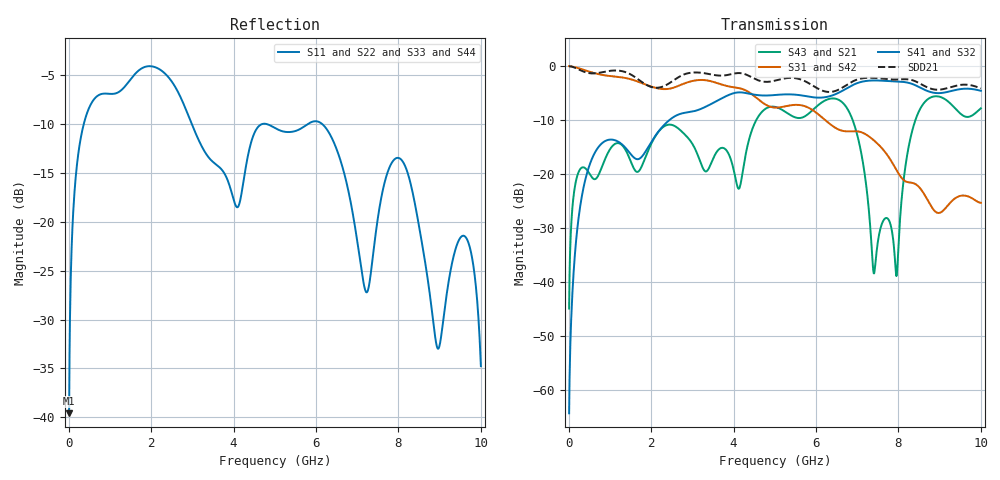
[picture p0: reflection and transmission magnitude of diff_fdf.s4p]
# HZ S RI R 50
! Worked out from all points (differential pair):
!   1000 points, 10 MHz to 10 GHz, reference 50 ohm
!   strongest paths, dB at 10 MHz, 2.51 GHz, 5.01 GHz, 7.51 GHz, 10 GHz:
!     S41: -64.4, -9.6, -5.4, -2.7, -4.6
!     S32: -64.4, -9.6, -5.4, -2.7, -4.6
!     S31: 0.0, -4.1, -7.7, -14.5, -25.3
!     S42: 0.0, -4.1, -7.7, -14.5, -25.3
!     S43: -44.9, -10.9, -7.6, -32.1, -7.8
!     S21: -44.9, -10.9, -7.6, -32.1, -7.8
!   taken as a pair (ports 1,2 in; 3,4 out), SDD21 dB: 0.0, -2.8, -2.7, -2.2, -4.2
!   lowest |S11| = -39.6 dB at 10 MHz (marker M1), VSWR 1.02, Z = 49.9 - j1.05 ohm
!   |S11| at or under -10 dB: 2.984 GHz to 4.713 GHz (1.729 GHz wide, 44.9 % of centre); 4.779 GHz to 5.807 GHz (1.028 GHz wide, 19.4 % of centre); 6.145 GHz to end of sweep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
1e7  -0.000638 -0.0105  0.000355 0.00565  0.9982 -0.0423  9.46e-05 -0.000597
     0.000355 0.00565  -0.000638 -0.0105  9.46e-05 -0.000597  0.9982 -0.0423
     0.9982 -0.0423  9.46e-05 -0.000597  -0.000638 -0.0105  0.000355 0.00565
     9.46e-05 -0.000597  0.9982 -0.0423  0.000355 0.00565  -0.000638 -0.0105
8.4e8  0.1036 0.4391  0.1207 0.0352  -0.8111 0.1555  0.0712 0.184
       0.1207 0.0352  0.1036 0.4391  0.0712 0.184  -0.8111 0.1555
       -0.8111 0.1555  0.0712 0.184  0.1036 0.4391  0.1207 0.0352
       0.0712 0.184  -0.8111 0.1555  0.1207 0.0352  0.1036 0.4391
1.58e9  0.0226 -0.5593  -0.0871 -0.0716  0.7383 0.0631  -0.041 -0.1363
        -0.0871 -0.0716  0.0226 -0.5593  -0.041 -0.1363  0.7383 0.0631
        0.7383 0.0631  -0.041 -0.1363  0.0226 -0.5593  -0.0871 -0.0716
        -0.041 -0.1363  0.7383 0.0631  -0.0871 -0.0716  0.0226 -0.5593
2.47e9  -0.0181 0.5306  0.2865 0.0093  -0.6203 -0.0131  0.00072 0.3223
        0.2865 0.0093  -0.0181 0.5306  0.00072 0.3223  -0.6203 -0.0131
        -0.6203 -0.0131  0.00072 0.3223  -0.0181 0.5306  0.2865 0.0093
        0.00072 0.3223  -0.6203 -0.0131  0.2865 0.0093  -0.0181 0.5306
7.29e9  0.0343 -0.0332  -0.0406 -0.0131  -0.2222 -0.00121  0.039 0.7326
        -0.0406 -0.0131  0.0343 -0.0332  0.039 0.7326  -0.2222 -0.00121
        -0.2222 -0.00121  0.039 0.7326  0.0343 -0.0332  -0.0406 -0.0131
        0.039 0.7326  -0.2222 -0.00121  -0.0406 -0.0131  0.0343 -0.0332
7.94e9  -0.195 -0.0803  0.00165 -0.0119  0.0915 0.0625  0.2828 -0.6641
        0.00165 -0.0119  -0.195 -0.0803  0.2828 -0.6641  0.0915 0.0625
        0.0915 0.0625  0.2828 -0.6641  -0.195 -0.0803  0.00165 -0.0119
        0.2828 -0.6641  0.0915 0.0625  0.00165 -0.0119  -0.195 -0.0803
1e10  0.00364 0.0179  -0.025 0.4057  0.0208 0.0499  -0.5844 -0.0846
      -0.025 0.4057  0.00364 0.0179  -0.5844 -0.0846  0.0208 0.0499
      0.0208 0.0499  -0.5844 -0.0846  0.00364 0.0179  -0.025 0.4057
      -0.5844 -0.0846  0.0208 0.0499  -0.025 0.4057  0.00364 0.0179
